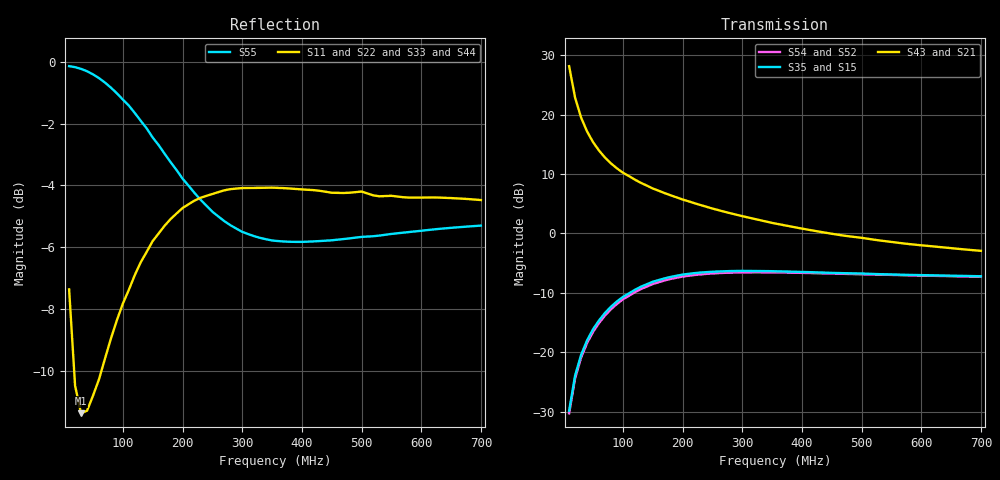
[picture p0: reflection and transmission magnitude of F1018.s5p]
! Date: Fri Aug 11 10:19:49 1995
!  POLYFET RF DEVICES
!  F1018 (Each Side)
!  S PARAMETERS
!  VDS=28V, IDQ=600mA
!AWR Design Environment (2053) Wed Feb 04 14:31:41 2004
!freq-unit  param-type  data-format  keyword  impedance-ohms
# MHz  S  MA  R  50
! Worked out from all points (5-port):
!   70 points, 10 MHz to 700 MHz, reference 50 ohm
!   strongest paths, dB at 10 MHz, 180 MHz, 360 MHz, 530 MHz, 700 MHz:
!     S43: 28.1, 6.4, 1.6, -1.2, -2.9
!     S21: 28.1, 6.4, 1.6, -1.2, -2.9
!     S35: -29.8, -7.3, -6.4, -6.8, -7.2
!     S15: -29.8, -7.3, -6.4, -6.8, -7.2
!     S54: -30.2, -7.6, -6.6, -6.9, -7.3
!     S52: -30.2, -7.6, -6.6, -6.9, -7.3
!   lowest |S11| = -11.4 dB at 30 MHz (marker M1), VSWR 1.74, Z = 51.2 - j28.4 ohm
!   |S11| at or under -10 dB: 18.49 MHz to 64.01 MHz (45.53 MHz wide, 110 % of centre)
